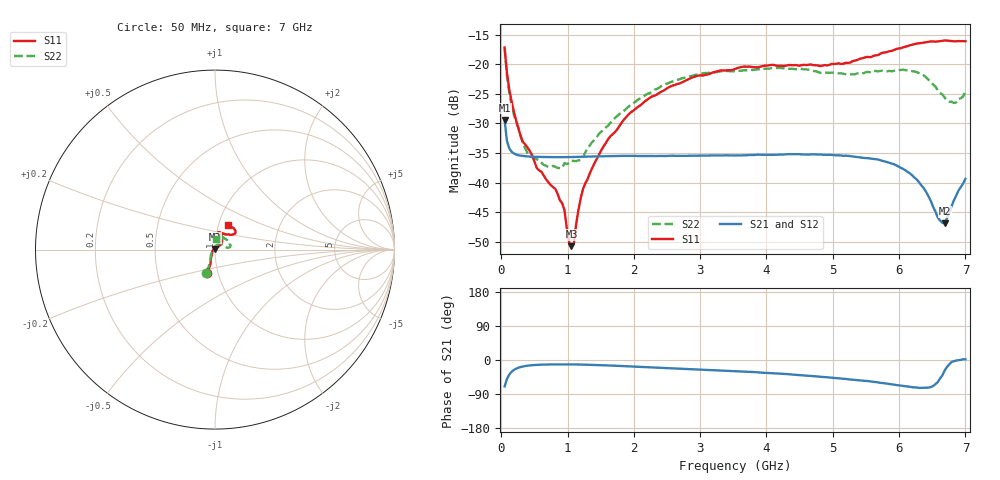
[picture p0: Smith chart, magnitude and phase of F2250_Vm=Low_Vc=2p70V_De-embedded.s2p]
! Integrated Device Technology
! Corporate Headquarters
! 6024 Silver Creek Valley Road
! San Jose, CA 95138  USA
! Phone:  1-408-284-8200
! Toll Free:  1-800-223-1366
! Webpage:  http://www.idt.com/
! Timing and RF Division
! 515 Groton Road, Suite 102
! Westford, MA 01886-6024
! Device:  F2250
! Description: Voltage Variable RF Attenuator
! Frequency:  50.0 -  6000.00 MHz
! Package:  3x3 mm Thin QFN Plastic Package: 16 pin
! Ports:  2 RF, 3 DC
!  Pin  1  = GND
!  Pin  2  = NC
!  Pin  3  = RF1  = Port 1
!  Pin  4  = NC
!  Pin  5  = GND
!  Pin  6  = GND
!  Pin  7  = GND
!  Pin  8  = GND
!  Pin  9  = NC
!  Pin 10  = RF2  = Port 2
!  Pin 11  = NC
!  Pin 12  = GND
!  Pin 13  = GND
!  Pin 14  = VCNTRL
!  Pin 15  = VDD
!  Pin 16  = VMODE
! Vcntrl:  2.700 Volts
! Vmode:  +0.000 Volts
! Vdd:  +3.30  Volts
! Current:  1.175 mA
! Data:  The device was measured on a the F2250 evaluation board which has
!  individual transmission lines to the RF pins.  Data was collected
!  using a calibrated network analyzer.  The evaluation board was
!  de-embedded using a TRL calibration technique.
!  The reference plane is the edge of the package pin.
! Misc:  SN 10
!  Action Tracker AT0258
! Date Measured:  2014-11-26
! Date:  2015-10-15  MJV
! Note:
!  Integrated Device Technology supplies this data as a sample of measured
!  data at the package pin for this product.  Your particular data for this
!  product may vary.
!  Data was taken at 25 degrees C.
!  Integrated Device Technology reserves the right to change this data at anytime.
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# GHz S dB R 50
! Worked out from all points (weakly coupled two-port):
!   201 points, 50 MHz to 7 GHz, reference 50 ohm
!   highest |S21| = -29.41 dB at 50 MHz (marker M1); lowest = -46.9 dB at 6.687 GHz (marker M2)
!   lowest |S11| = -50.7 dB at 1.058 GHz (marker M3), VSWR 1.01, Z = 49.8 + j0.243 ohm
!   |S11| at or under -10 dB: start of sweep to end of sweep
!   |S22| runs from -37.5 to -17.3 dB; largest |S21 - S12| = 6.2e-05
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0.05  -17.18 -108.6  -29.41 -69.8  -29.41 -69.8  -17.28 -111.0
0.08475  -21.45 -107.5  -32.92 -50.4  -32.92 -50.4  -21.75 -110.2
0.15425  -26.23 -116.6  -34.76 -31.1  -34.76 -31.1  -26.82 -122.4
0.29325  -32.21 -127.9  -35.43 -18.5  -35.43 -18.5  -32.09 -137.5
0.3975  -34.09 -141.9  -35.56 -15.0  -35.56 -15.0  -35.05 -160.5
0.91875  -43.48 158.2  -35.69 -11.5  -35.68 -11.5  -37.52 133.5
0.9535  -44.63 170.0  -35.68 -11.5  -35.69 -11.5  -36.67 131.3
1.023  -50.00 143.5  -35.67 -11.6  -35.67 -11.6  -36.66 115.9
1.05775  -50.70 123.3  -35.67 -11.6  -35.67 -11.6  -36.29 110.7
1.0925  -50.37 89.3  -35.66 -11.7  -35.66 -11.7  -36.32 106.3
1.162  -44.70 56.8  -35.64 -11.9  -35.64 -11.9  -36.22 95.6
1.2315  -41.09 44.3  -35.61 -12.1  -35.61 -12.1  -35.80 85.9
1.6485  -32.12 42.0  -35.52 -14.6  -35.52 -14.7  -29.87 64.6
1.9265  -28.39 41.3  -35.47 -16.9  -35.46 -16.9  -27.09 56.7
2.37825  -24.87 47.3  -35.48 -20.3  -35.48 -20.3  -23.99 56.8
3.525  -20.79 72.5  -35.41 -29.5  -35.41 -29.5  -21.19 74.8
4.7065  -20.17 72.3  -35.20 -42.5  -35.20 -42.6  -21.14 72.3
5.85325  -17.81 40.5  -36.64 -63.3  -36.64 -63.4  -21.13 23.0
6.27025  -16.50 40.1  -39.49 -72.7  -39.50 -72.7  -21.36 9.7
6.68725  -15.99 48.8  -46.86 -27.8  -46.81 -27.2  -25.63 28.5
6.861  -16.13 55.1  -42.18 -1.3  -42.15 -1.3  -26.46 57.9
7  -16.13 63.2  -39.35 1.9  -39.30 1.8  -24.63 83.1
